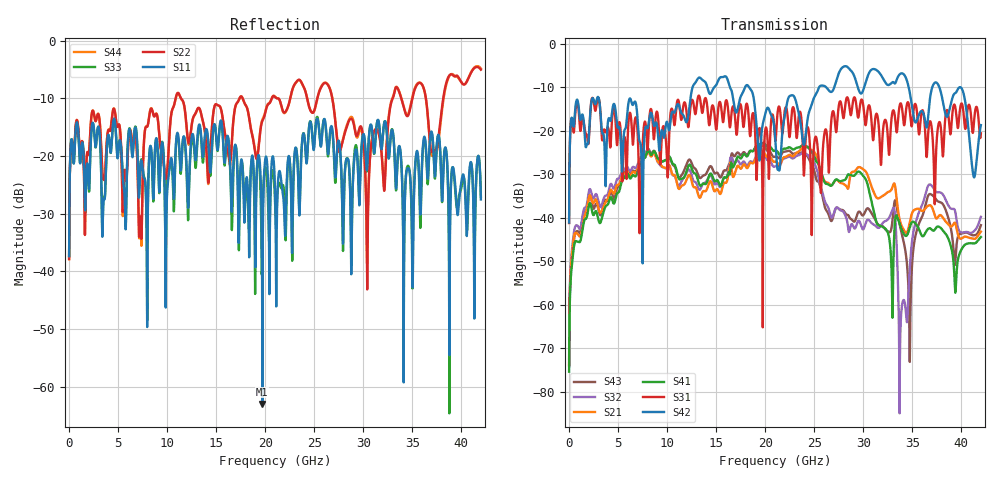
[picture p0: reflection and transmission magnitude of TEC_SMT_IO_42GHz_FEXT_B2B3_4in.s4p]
!! CHANNEL DESCRIPTION: Next Generation 28Gbps High Density SMT I/O Connector
!!  with 4" 5-6-5 Megatron 6 Stripline trace on host side and 1.25" 7-5-7 Megtron 6 Microstrip trace on plug side at 14GHz
!! HOST PCB DESCRIPTION: PCB thickness 2.86 mm, Nelco 4000-13SI (Dk 3.32, Df 0.010)
!!  23 Layer Board, 12 GND planes, 2 Layer route-out on Layers 10,12, 8 mil stub on vias
!!  Pairs on following layers
!!  Layer 10 - B2B3
!! CONNECTOR DESCRIPTION:  Next Generation 28Gbps High Density SMT I/O Connector
!! PLUG-IN CARD DESCRIPTION:  PCB thickness 1mm thick, Nelco 4000-13SI (Dk 3.32, Df 0.010)
!!  6 Layer Board, 4 GND planes, 0.35 x 1.4mm mating pads
!!  Micro-strip diff traces referenced to GND plane 3mils down, 2nd GND plane 15mils from top of board
!!  PCB GND planes are symmetric
!! MODEL DESCRIPTION: TE Connectivity S-parameter model produced from Macro-model
!! MODEL DATE: 9/25/2014 CR1a_GC1i, VR6&12_4
!! MODEL STATUS: Developmental
!! MODEL GEOMETRY: 2 Rows - Rows A, B. 3 pairs in each row, 6 total pairs
!! MODEL FREQUENCY RANGE: DC to 42 GHz in 10 MHz frequency steps
!! MODEL EDGE RATE LIMITATION: 11.90 ps (Using conservative 0.5/Fmax rule of thumb)
!! TIME-DOMAIN TRANSFORM CAUTIONS:
!! 1.) Do not simulate transient edge rates faster than the number listed above.  Edge
!!  rates faster than this number contain significant spectral content at frequencies
!!  above the model's highest frequency.
!! 2.) Even when simulating edge rates that are slower than the number listed above, be
!!  aware that the best time resolution possible with a direct iFFT is (1 / 2Fmax).
!!  As a result, time resolution is typically not adequate for most time-domain
!!  simulations unless tricks such as frequency-domain zero-padding and windowing are
!!  used to minimize leakage and aliasing.
!! 3.) Because the model has a uniform frequency step, a direct iFFT will result in an
!!  impulse that that has a time length given by either (1 / Fstep) or (1 / 2Fstep),
!!  depending on the transform being used.  Care has been taken in selecting the
!!  frequency step to ensure a settled impulse response for the model.  Therefore,
!!  convolution with the model's impulse response should present no issues.  However,
!!  if directly concatenating s-parameter models in the frequency domain a user must
!!  either interpolate necessary interim frequencies or complete impulse response
!!  zero-padding.  Impulse response zero-padding is more difficult, but more accurate.
!! PORT DEFINITIONS:
!! Port  1  ----->  Host, Bot Row  B2  B5  Module, Top Row  <-----  Port  2
!! Port  3  ----->  Host, Bot Row  B3  B6  Module, Top Row  <-----  Port  4
# Hz S MA R 50
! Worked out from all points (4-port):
!   4200 points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, 10 MHz to 42 GHz, reference 50 ohm
!   strongest paths, dB at 10 MHz, 10.51 GHz, 21.01 GHz, 31.51 GHz, 42 GHz:
!     S42: -41.1, -15.7, -21.2, -6.3, -18.7
!     S31: -41.2, -15.0, -21.8, -17.3, -20.6
!     S41: -75.4, -27.3, -24.6, -41.6, -44.4
!     S21: -73.8, -29.9, -27.1, -35.5, -43.2
!     S32: -72.5, -30.0, -28.2, -42.3, -39.8
!     S43: -74.0, -27.5, -25.9, -41.5, -41.7
!   lowest |S11| = -62.9 dB at 19.71 GHz (marker M1), VSWR 1.00, Z = 49.9 - j0.0274 ohm
!   |S11| at or under -10 dB: start of sweep to end of sweep
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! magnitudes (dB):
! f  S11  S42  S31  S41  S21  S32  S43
! 10 MHz  -37.3  -41.1  -41.2  -75.4  -73.8  -72.5  -74.0
! 2.12 GHz  -22.3  -17.5  -17.5  -36.6  -34.8  -33.4  -34.9
! 19.71 GHz  -62.9  -19.1  -31.9  -22.8  -25.3  -25.5  -23.4
! 33.06 GHz  -16.3  -8.8  -15.3  -52.3  -32.5  -37.8  -38.9
! 33.81 GHz  -19.4  -6.9  -13.7  -42.1  -41.2  -64.9  -42.5
! 36.66 GHz  -21.8  -15.8  -19.6  -42.5  -37.2  -32.5  -34.8
! 42 GHz  -27.5  -18.7  -20.6  -44.4  -43.2  -39.8  -41.7
